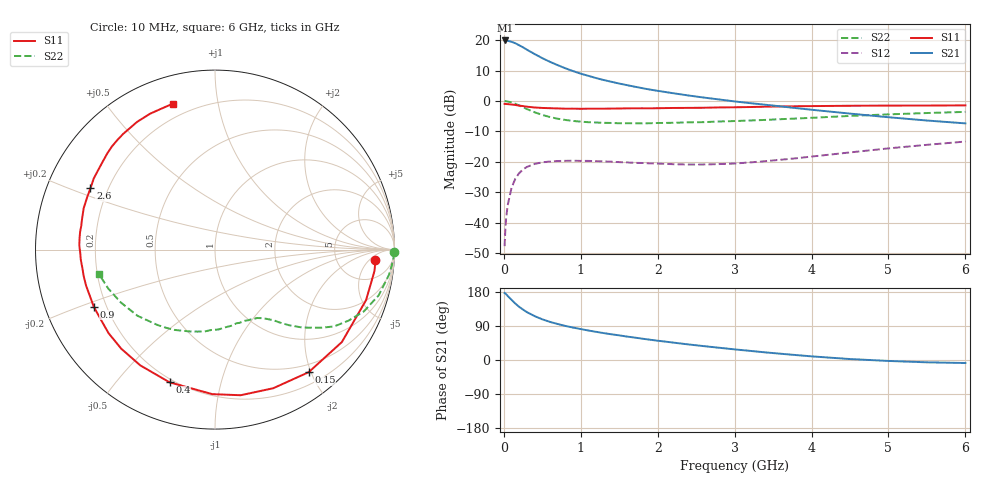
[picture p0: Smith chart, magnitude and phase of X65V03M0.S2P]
! SIEMENS Small Signal Semiconductors
! BFP193W
! Si NPN RF Bipolar Junction Transistor in SOT343
! VCE = 5 V  IC = 3 mA
! Common Emitter S-Parameters:  April 1994
# GHz  S  MA  R  50
!  f  S11  S21  S12  S22
! GHz  MAG  ANG  MAG  ANG  MAG  ANG  MAG  ANG
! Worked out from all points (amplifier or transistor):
!   40 points, 10 MHz to 6 GHz, reference 50 ohm
!   highest |S21| = 19.9 dB at 20 MHz (marker M1)
!   |S21| within 3 dB of that: start of sweep to 297.4 MHz
!   unconditionally stable (mu >= 1): 1.946 GHz to 4.507 GHz
!   at 200 MHz: K = 0.11, MSG = 21.0 dB, |S12| = -23.7 dB
!   at 1.5 GHz: K = 0.77, MSG = 12.9 dB, |S12| = -20.1 dB
!   at 6 GHz: K = 0.94, MSG = 3.0 dB, |S12| = -13.3 dB
!   S11 on the Smith chart (normalised r, x): 10 MHz: 14, -8; 150 MHz: 0.38, -1.97; 400 MHz: 0.18, -0.70; 900 MHz: 0.15, -0.22; 2.6 GHz: 0.13, +0.23; 6 GHz: 0.13, +0.75
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0.01  0.8959 -3.6  9.834 177.0  0.0041 88.9  0.9999 -0.9
0.02  0.8966 -7.5  9.878 175.6  0.0079 87.7  0.9932 -3.5
0.05  0.8875 -18.5  9.758 169.1  0.0193 79.5  0.98 -8.2
0.1  0.8746 -36.1  9.389 158.7  0.0373 70.7  0.9469 -15.6
0.15  0.8596 -52.6  8.883 148.8  0.0529 62.1  0.8983 -22.5
0.2  0.8378 -67.2  8.223 140.2  0.0652 54.6  0.8428 -28.0
0.25  0.8239 -80.0  7.614 133.0  0.0751 48.4  0.79 -32.8
0.3  0.8054 -91.1  6.961 126.3  0.0824 43.1  0.7355 -36.3
0.4  0.7816 -108.9  5.906 115.8  0.0923 34.7  0.6514 -41.8
0.5  0.7677 -122.8  5.057 107.3  0.098 28.8  0.5899 -45.6
0.6  0.7601 -133.4  4.392 100.5  0.1011 24.3  0.5436 -48.4
0.7  0.754 -141.9  3.881 95.0  0.103 21.1  0.5104 -50.4
0.9  0.7467 -154.8  3.101 85.5  0.1041 16.5  0.4694 -54.6
1.1  0.7458 -164.3  2.586 77.8  0.1034 13.6  0.4473 -58.4
1.3  0.7462 -172.4  2.206 70.9  0.1015 12.0  0.4372 -62.7
1.6  0.7565 178.2  1.82 61.8  0.0977 11.8  0.4301 -68.9
2.2  0.7669 162.6  1.341 46.0  0.0913 16.0  0.4374 -82.9
2.6  0.7733 153.8  1.137 36.6  0.0903 22.0  0.4485 -92.7
3.2  0.7945 142.0  0.921 24.1  0.0976 31.8  0.4772 -107.2
4.5  0.8336 121.3  0.62 2.5  0.1426 42.6  0.5679 -139.5
5.5  0.8402 110.8  0.477 -6.1  0.1901 40.5  0.6333 -160.0
6  0.8462 106.0  0.428 -8.0  0.2151 38.3  0.6616 -168.3
